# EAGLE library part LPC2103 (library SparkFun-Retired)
NXP LPC2103 ARM7 based MCU Dead prototype
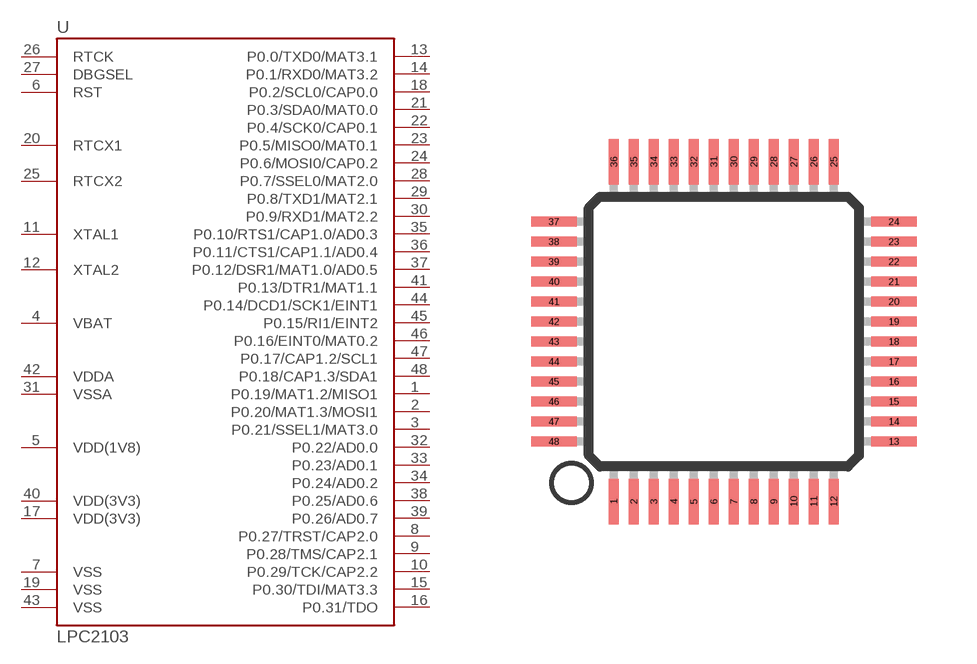
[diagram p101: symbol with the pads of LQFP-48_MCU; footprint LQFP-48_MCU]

Designator prefix -

## LPC2103 (PROD_ID: IC-09387; VALUE: LPC2103)  [LQFP-48_MCU]
1  P0.19/MAT1.2/MISO1
2  P0.20/MAT1.3/MOSI1
3  P0.21/SSEL1/MAT3.0
4  VBAT
5  VDD(1V8)
6  RST
7  VSS
8  P0.27/TRST/CAP2.0
9  P0.28/TMS/CAP2.1
10  P0.29/TCK/CAP2.2
11  XTAL1
12  XTAL2
13  P0.0/TXD0/MAT3.1
14  P0.1/RXD0/MAT3.2
15  P0.30/TDI/MAT3.3
16  P0.31/TDO
17  VDD(3V3)
18  P0.2/SCL0/CAP0.0
19  VSS
20  RTCX1
21  P0.3/SDA0/MAT0.0
22  P0.4/SCK0/CAP0.1
23  P0.5/MISO0/MAT0.1
24  P0.6/MOSI0/CAP0.2
25  RTCX2
26  RTCK
27  DBGSEL
28  P0.7/SSEL0/MAT2.0
29  P0.8/TXD1/MAT2.1
30  P0.9/RXD1/MAT2.2
31  VSSA
32  P0.22/AD0.0
33  P0.23/AD0.1
34  P0.24/AD0.2
35  P0.10/RTS1/CAP1.0/AD0.3
36  P0.11/CTS1/CAP1.1/AD0.4
37  P0.12/DSR1/MAT1.0/AD0.5
38  P0.25/AD0.6
39  P0.26/AD0.7
40  VDD(3V3)
41  P0.13/DTR1/MAT1.1
42  VDDA
43  VSS
44  P0.14/DCD1/SCK1/EINT1
45  P0.15/RI1/EINT2
46  P0.16/EINT0/MAT0.2
47  P0.17/CAP1.2/SCL1
48  P0.18/CAP1.3/SDA1

## Footprint LQFP-48_MCU (pad centres in mm)
smd 0.254 x 1.143: 1 -2.75,-4.25; 2 -2.25,-4.25; 3 -1.75,-4.25; 4 -1.25,-4.25; 5 -0.75,-4.25; 6 -0.25,-4.25; 7 0.25,-4.25; 8 0.75,-4.25; 9 1.25,-4.25; 10 1.75,-4.25; 11 2.25,-4.25; 12 2.75,-4.25; 25 2.75,4.25; 26 2.25,4.25; 27 1.75,4.25; 28 1.25,4.25; 29 0.75,4.25; 30 0.25,4.25; 31 -0.25,4.25; 32 -0.75,4.25; 33 -1.25,4.25; 34 -1.75,4.25; 35 -2.25,4.25; 36 -2.75,4.25
smd 1.143 x 0.254: 13 4.25,-2.75; 14 4.25,-2.25; 15 4.25,-1.75; 16 4.25,-1.25; 17 4.25,-0.75; 18 4.25,-0.25; 19 4.25,0.25; 20 4.25,0.75; 21 4.25,1.25; 22 4.25,1.75; 23 4.25,2.25; 24 4.25,2.75; 37 -4.25,2.75; 38 -4.25,2.25; 39 -4.25,1.75; 40 -4.25,1.25; 41 -4.25,0.75; 42 -4.25,0.25; 43 -4.25,-0.25; 44 -4.25,-0.75; 45 -4.25,-1.25; 46 -4.25,-1.75; 47 -4.25,-2.25; 48 -4.25,-2.75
